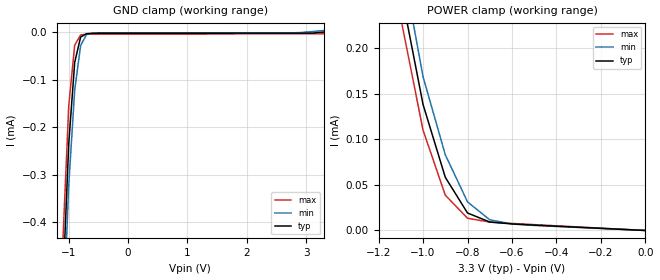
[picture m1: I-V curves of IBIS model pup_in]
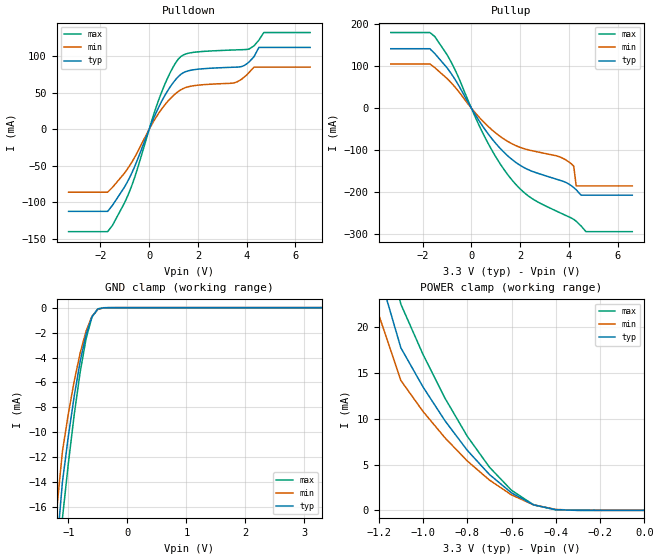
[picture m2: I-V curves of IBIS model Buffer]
| IBIS file EG2002_H.ibs
[IBIS ver]   2.1
[File name]   eg2002_h.ibs
[File Rev]   2
[Date]   December 26, 2006
[Source]   This file is for EG2002CA PC parts.
[Notes]   File generated by ms.
[Disclaimer]   This information is for modeling purposes only and is not
   guaranteed.
|   Component EG-2002CA (125.0 - 170.0MHz)
[Component]   EG-2002CA
[Manufacturer] Epson Toyocom Corp.
[Package]
| variable   typ   min   max
R_pkg   0.78   NA   NA
L_pkg   2.19nH   NA   NA
C_pkg   3.99pF   NA   NA
[Pin]  signal_name   model_name   R_pin   L_pin   C_pin
1   oe   pup_in   NA   NA   NA
2   vss   GND   NA   NA   NA
3   out   Buffer   NA   NA   NA
4   vdd   POWER   NA   NA   NA
| Models and submodels in the file (2): pup_in (Input), Buffer (3-state)
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|   Model pup_in
[Model]   pup_in
Model_type   Input
C_comp   0.00pF  0.00pF  0.00pF
Vinl =   0.6600V
Vinh =   2.6400V
[Temperature Range]   25.0000   70.0000   0.0000
[Voltage Range]   3.3000V   3.0000V   3.6000V
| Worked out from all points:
|   GND clamp passes 1 mA (typ) near -1.15 V on its own axis
|   POWER clamp passes 1 mA (typ) near -1.19 V on its own axis
[GND_clamp]
| voltage   I(typ)   I(min)   I(max)
-1.3V     -31.7mA    -18.35mA   -67.82mA
-1.1V     -533.4uA   -626.3uA   -441.4uA
-1V       -233.7uA   -320.7uA   -154.2uA
-900mV    -63.74uA   -121.8uA   -27.65uA
-800mV    -10.47uA   -28.19uA   -5.886uA
-700mV    -3.32uA    -5.252uA   -4.357uA
-600mV    -2.697uA   -2.031uA   -4.278uA
2.8V      -2.21uA    -1.38uA    -3.51uA
3.1V      -2.21uA    1.093uA    -3.51uA
3.3V      13.2pA     3.295uA    -3.51uA
[POWER_clamp]
| voltage   I(typ)   I(min)   I(max)
-1.3V     32.03mA    18.21mA    82.7mA
-1.1V     263.5uA    301.8uA    232.4uA
-1V       138.1uA    168.5uA    110uA
-900mV    58.31uA    83.05uA    38.69uA
-800mV    19.15uA    31.29uA    13.42uA
-700mV    9.289uA    11.71uA    9.178uA
-600mV    7.144uA    7.117uA    7.697uA
0V        13.2pA     12.01pA    14.4pA
|   Model Buffer
[Model]   Buffer
Model_type   3-state
Polarity   Non-Inverting
Enable   Active-High
C_comp   0.00pF   0.00pF   0.00pF
[Temperature Range]   25.00   70.00   0.00
[Voltage Range]   3.30V   3.00V   3.60V
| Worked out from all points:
|   slope of the pulldown table from 0 to 0.495 V, typ, clamps not added: 13.3 ohm
|   slope of the pullup table from 0 to 0.495 V, typ, clamps not added: 10.9 ohm
|   GND clamp passes 1 mA (typ) near -0.62 V on its own axis
|   POWER clamp passes 1 mA (typ) near -0.53 V on its own axis
[Pulldown]
|voltage I(typ)   I(min)   I(max)
-3.3V     -112.2mA   -86.01mA   -140mA
-1.7V     -112.2mA   -86.01mA   -140mA
-1.5V     -103.9mA   -79.31mA   -131.3mA
-700mV    -59.06mA   -44.43mA   -76.01mA
200mV     16.4mA     11.98mA    21.73mA
600mV     43.86mA    31.86mA    58.36mA
1.3V      75.5mA     54.35mA    99.86mA
3.8V      86.26mA    69.1mA     109.3mA
4.3V      99.66mA    85.45mA    114.6mA
4.5V      112.4mA    85.45mA    122.3mA
4.7V      112.4mA    85.45mA    132.8mA
6.6V      112.4mA    85.45mA    132.8mA
[Pullup]
|voltage I(typ)   I(min)   I(max)
-3.3V     141.4mA    105.1mA    180mA
-1.7V     141.4mA    105.1mA    180mA
-1.5V     130.1mA    96.4mA     170.7mA
-800mV    80.1mA     58.69mA    106.7mA
900mV     -77.15mA   -54.69mA   -106.2mA
1.6V      -119.4mA   -83.07mA   -166.7mA
2.2V      -143.1mA   -97.57mA   -203.2mA
4V        -181.2mA   -128.5mA   -259.5mA
4.2V      -189.7mA   -138.8mA   -265.5mA
4.3V      -194.8mA   -185.7mA   -269.9mA
4.7V      -207.7mA   -185.7mA   -294.7mA
6.6V      -207.7mA   -185.7mA   -294.7mA
[GND_clamp]
|voltage   I(typ)   I(min)   I(max)
-1.3V     -100.2mA   -61.96mA   -197.5mA
-1.2V     -19.54mA   -16.36mA   -23.33mA
-1.1V     -13.98mA   -11.53mA   -16.89mA
-1V       -10.32mA   -8.51mA    -12.51mA
-900mV    -7.084mA   -5.883mA   -8.571mA
-800mV    -4.329mA   -3.651mA   -5.184mA
-700mV    -2.159mA   -1.887mA   -2.505mA
-600mV    -723.6uA   -694.4uA   -756.6uA
-500mV    -118.1uA   -141.8uA   -93.45uA
-400mV    -9.354uA   -15.45uA   -5.252uA
-300mV    -724.3nA   -1.444uA   -402.3nA
3.3V      53.74pA    6.845uA    46.58pA
[POWER_clamp]
|voltage   I(typ)   I(min)   I(max)
-1.3V     206.5mA    121.8mA    427.3mA
-1.2V     26.05mA    21.37mA    32.5mA
-1.1V     17.75mA    14.19mA    22.52mA
-1V       13.49mA    10.81mA    17.04mA
-900mV    9.763mA    7.908mA    12.22mA
-800mV    6.559mA    5.398mA    8.096mA
-700mV    3.92mA     3.31mA     4.723mA
-600mV    1.905mA    1.688mA    2.187mA
-500mV    599.8uA    597.2uA    601.2uA
-400mV    75.4uA     101.1uA    51.08uA
-300mV    3.37uA     6.845uA    1.412uA
0V        53.74pA    68.56pA    57.62pA
[Ramp]
| variable   typ   min   max
dV/dt_r   1.6217/0.2273n   1.3661/0.2956n   1.8641/0.1805n
dV/dt_f   1.5414/0.3078n   1.2673/0.4084n   1.7902/0.2399n
R_load = 50.0000
| End [Model] Buffer
| End [Component] EG-2002CA
